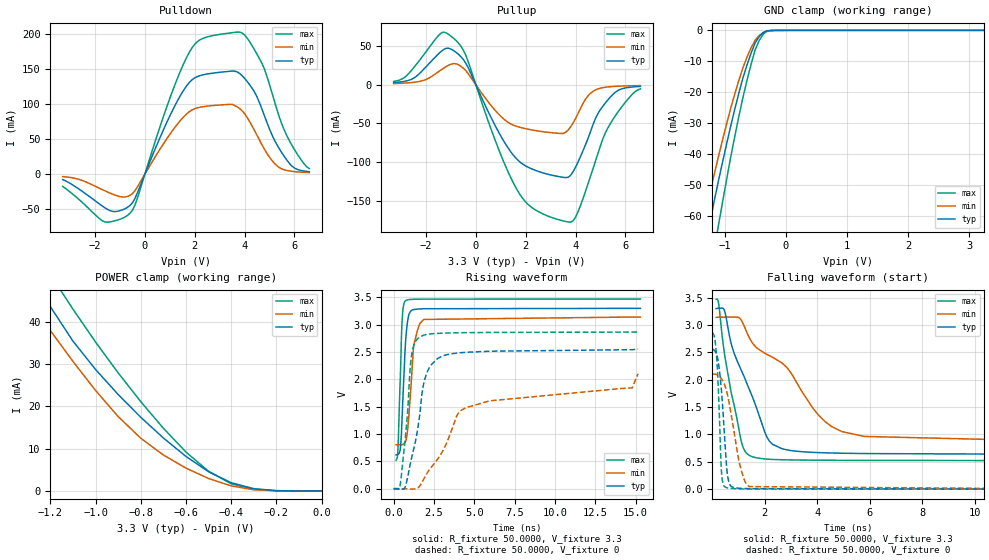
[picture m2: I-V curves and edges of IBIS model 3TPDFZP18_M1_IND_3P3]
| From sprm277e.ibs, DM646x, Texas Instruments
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|   Model Cell 3TPDFZP18_M1_IND_3P3
|BPCI33TPDFZP18_M1_IND_3P3
[Model]   3TPDFZP18_M1_IND_3P3
Model_type   I/O
Polarity   Non-Inverting
Enable   Active-Low
Vinl =  0.99V
Vinh =  1.65V
Cref =  10.0000pF
Rref =  50.0000
Vref =  1.5V
Vmeas =  1.65
C_comp   3.400798p   3.348868p   3.529696p
[Model Spec]
Vinl   0.99V   0.942V   1.041V
Vinh   1.65V   1.570V   1.735V
[Temperature Range]   25   125   -40
[Voltage Range]   3.3   3.14   3.47
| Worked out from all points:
|   slope of the pulldown table from 0 to 0.495 V, typ, clamps not added: 11.5 ohm
|   slope of the pullup table from 0 to 0.495 V, typ, clamps not added: 14.2 ohm
|   GND clamp passes 1 mA (typ) near -0.38 V on its own axis
|   POWER clamp passes 1 mA (typ) near -0.33 V on its own axis
|   rising waveform, R_fixture 50.0000, V_fixture 3.3: 20-80 % time 256ps typ, 353ps min, 184ps max; typ from 0.619 V to 3.3 V
|   rising waveform, R_fixture 50.0000, V_fixture 0: 20-80 % time 902ps typ, 6.24ns min, 456ps max; typ from 0 V to 2.56 V
|   falling waveform, R_fixture 50.0000, V_fixture 3.3: 20-80 % time 1.25ns typ, 2.7ns min, 650ps max; typ from 3.3 V to 0.619 V
|   falling waveform, R_fixture 50.0000, V_fixture 0: 20-80 % time 227ps typ, 466ps min, 142ps max; typ from 2.56 V to 0 V
[POWER_clamp]
|   voltage   I(typ)   I(min)   I(max)
-3.3V     266.8mA    199mA      322.6mA
-1.333V   56.66mA    48mA       64.27mA
-1.3V     53.18mA    45.44mA    60.44mA
-1.233V   46.77mA    40.42mA    54.26mA
-1.133V   38.14mA    33.06mA    45.71mA
-1V       28.71mA    23.76mA    35.2mA
-800mV    17.41mA    12.45mA    21.11mA
-600mV    8.154mA    5.386mA    9.19mA
-500mV    4.533mA    2.939mA    4.641mA
-400mV    1.938mA    1.191mA    1.687mA
-300mV    534.7uA    277uA      402uA
0V        182.2nA    556.5nA    317.7nA
[Pulldown]
|   voltage   I(typ)   I(min)   I(max)
-3.3V     -7.788mA   -3.439mA   -17.46mA
-1.6V     -48.12mA   -23.82mA   -68.34mA
-600mV    -44.86mA   -30.4mA    -55.99mA
1V        83.15mA    56.86mA    108.2mA
1.8V      131.8mA    89.77mA    175.4mA
2.3V      141.8mA    96.35mA    193.8mA
3.7V      146.4mA    96.42mA    203.3mA
4.1V      132.9mA    81.48mA    194.9mA
4.7V      93.03mA    41.99mA    158.5mA
5.3V      42.12mA    11.99mA    92.47mA
5.9V      11.6mA     4.111mA    41.42mA
6.6V      3.544mA    2.265mA    7.965mA
[Pullup]
|   voltage   I(typ)   I(min)   I(max)
-3.3V     2.84mA     1.649mA    4.344mA
-2.5V     8.541mA    3.25mA     22.02mA
-1.4V     43.04mA    19.26mA    66.82mA
-1V       46.23mA    26.7mA     63mA
-400mV    27.63mA    18.2mA     37.7mA
900mV     -60.4mA    -37.48mA   -82.33mA
1.8V      -100.6mA   -55.19mA   -143.4mA
2.5V      -111.9mA   -59.72mA   -163.8mA
3.8V      -117mA     -54.41mA   -177.6mA
4.5V      -69.24mA   -14.23mA   -127.9mA
5.2V      -23.21mA   -3.139mA   -61.78mA
6.6V      -2.032mA   -953.4uA   -5.249mA
[GND_clamp]
|   voltage   I(typ)   I(min)   I(max)
-3.3V     -301.2mA   -227.6mA   -361.6mA
-1.367V   -75.5mA    -63.1mA    -93.47mA
-1.3V     -68.14mA   -57.39mA   -85.75mA
-1.233V   -61.34mA   -51.76mA   -78.08mA
-1.1V     -48.49mA   -40.68mA   -62.86mA
-833.3mV  -25.4mA    -20.48mA   -34.13mA
-633.3mV  -11.11mA   -8.597mA   -16.02mA
-500mV    -3.958mA   -3.124mA   -6.237mA
-366.7mV  -691.7uA   -679.4uA   -1.198mA
-300mV    -116.7uA   -170.2uA   -183.7uA
-166.7mV  -12.04uA   -19.37uA   -14.28uA
3.233V    119.2nA    5.035uA    262.1nA
[Ramp]
| variable   typ   min   max
dV/dt_f  1.6137532/1.2498139n  1.4059296/2.694372n   1.7744748/0.65132499n
dV/dt_r  1.5402618/0.90498157n   1.26697/5.2850635n   1.72403/0.45834663n
R_load = 50
[Rising Waveform]
R_fixture = 50.0000
V_fixture = 3.3
V_fixture_min = 3.14
V_fixture_max = 3.47
|   time   V(typ)   V(min)   V(max)
146.6ps   618.5mV    802.6mV    519.5mV
263.7ps   624.1mV    802.7mV    704.4mV
439.3ps   807.4mV    802.6mV    2.28V
498ps     1.121V     803.8mV    2.901V
559.5ps   1.557V     809.4mV    3.227V
745.7ps   2.715V     871.8mV    3.442V
933.2ps   3.173V     1.296V     3.459V
1.259ns   3.279V     2.64V      3.466V
1.866ns   3.293V     3.097V     3.469V
15.3ns    3.3V       3.14V      3.47V
[Rising Waveform]
R_fixture = 50.0000
V_fixture = 0
V_fixture_min = 0
V_fixture_max = 0
|   time   V(typ)   V(min)   V(max)
100.8fs   23.63uV    17.75uV    31.17uV
400.6ps   -3.037mV   15.66uV    60.56mV
780.2ps   94.33mV    -2.19mV    1.109V
1.099ns   548.2mV    -9.242mV   2.419V
1.624ns   1.364V     51.18mV    2.775V
1.861ns   1.92V      169.9mV    2.807V
2.309ns   2.261V     383mV      2.833V
4.455ns   2.495V     1.48V      2.855V
14.79ns   2.542V     1.844V     2.865V
15.15ns   2.557V     2.102V     2.867V
[Falling Waveform]
R_fixture = 50.0000
V_fixture = 3.3
V_fixture_min = 3.14
V_fixture_max = 3.47
|   time   V(typ)   V(min)   V(max)
146.6ps   3.3V       3.14V      3.47V
244.6ps   3.306V     3.142V     3.373V
448.4ps   3.278V     3.143V     2.524V
730.3ps   2.638V     3.145V     1.737V
1.094ns   2.182V     3.095V     893mV
1.485ns   1.736V     2.702V     600.7mV
2.302ns   817.9mV    2.41V      542.9mV
4.031ns   668.4mV    1.361V     529.4mV
4.936ns   656.9mV    1.053V     527.2mV
15.3ns    618.5mV    802.6mV    519.5mV
[Falling Waveform]
R_fixture = 50.0000
V_fixture = 0
V_fixture_min = 0
V_fixture_max = 0
|   time   V(typ)   V(min)   V(max)
100.8fs   2.557V     2.102V     2.867V
146.7ps   2.481V     2.097V     2.52V
265.6ps   2.187V     2.063V     1.367V
356.2ps   1.746V     2.011V     265mV
510.9ps   621.8mV    1.846V     32.93mV
583.6ps   234.6mV    1.709V     22.77mV
687.2ps   65mV       1.45V      15.94mV
1.048ns   15.96mV    445.2mV    4.748mV
1.412ns   9.487mV    47.16mV    1.838mV
15.15ns   23.63uV    17.75uV    31.17uV
